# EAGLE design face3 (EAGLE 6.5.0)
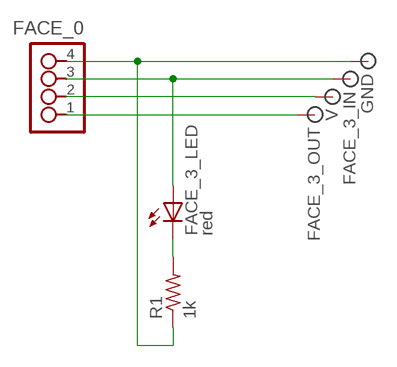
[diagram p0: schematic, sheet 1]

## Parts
FACE_0  4_PIN_HEADER  [SMT_PINS_4]
FACE_3_IN  SIGNAL  [PAD.2]
FACE_3_LED  red  LED1206  [1206]
FACE_3_OUT  SIGNAL  [PAD.2]
GND  SIGNAL  [PAD.2]
R1  1k  RESISTOR1206  [1206]
V  SIGNAL  [PAD.2]

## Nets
N$2: FACE_0.3 FACE_3_IN.P$1 FACE_3_LED.1(A)
N$3: FACE_0.2 V.P$1
N$4: FACE_0.1 FACE_3_OUT.P$1
N$5: FACE_3_LED.2(C) R1.2
N$6: FACE_0.4 GND.P$1 R1.1

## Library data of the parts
FACE_0 = ot:4_PIN_HEADER
FACE_3_IN FACE_3_OUT GND V = ot:SIGNAL: Signal
FACE_3_LED = 01_FAB_Hello:LED
R1 = 01_FAB_Hello:RESISTOR

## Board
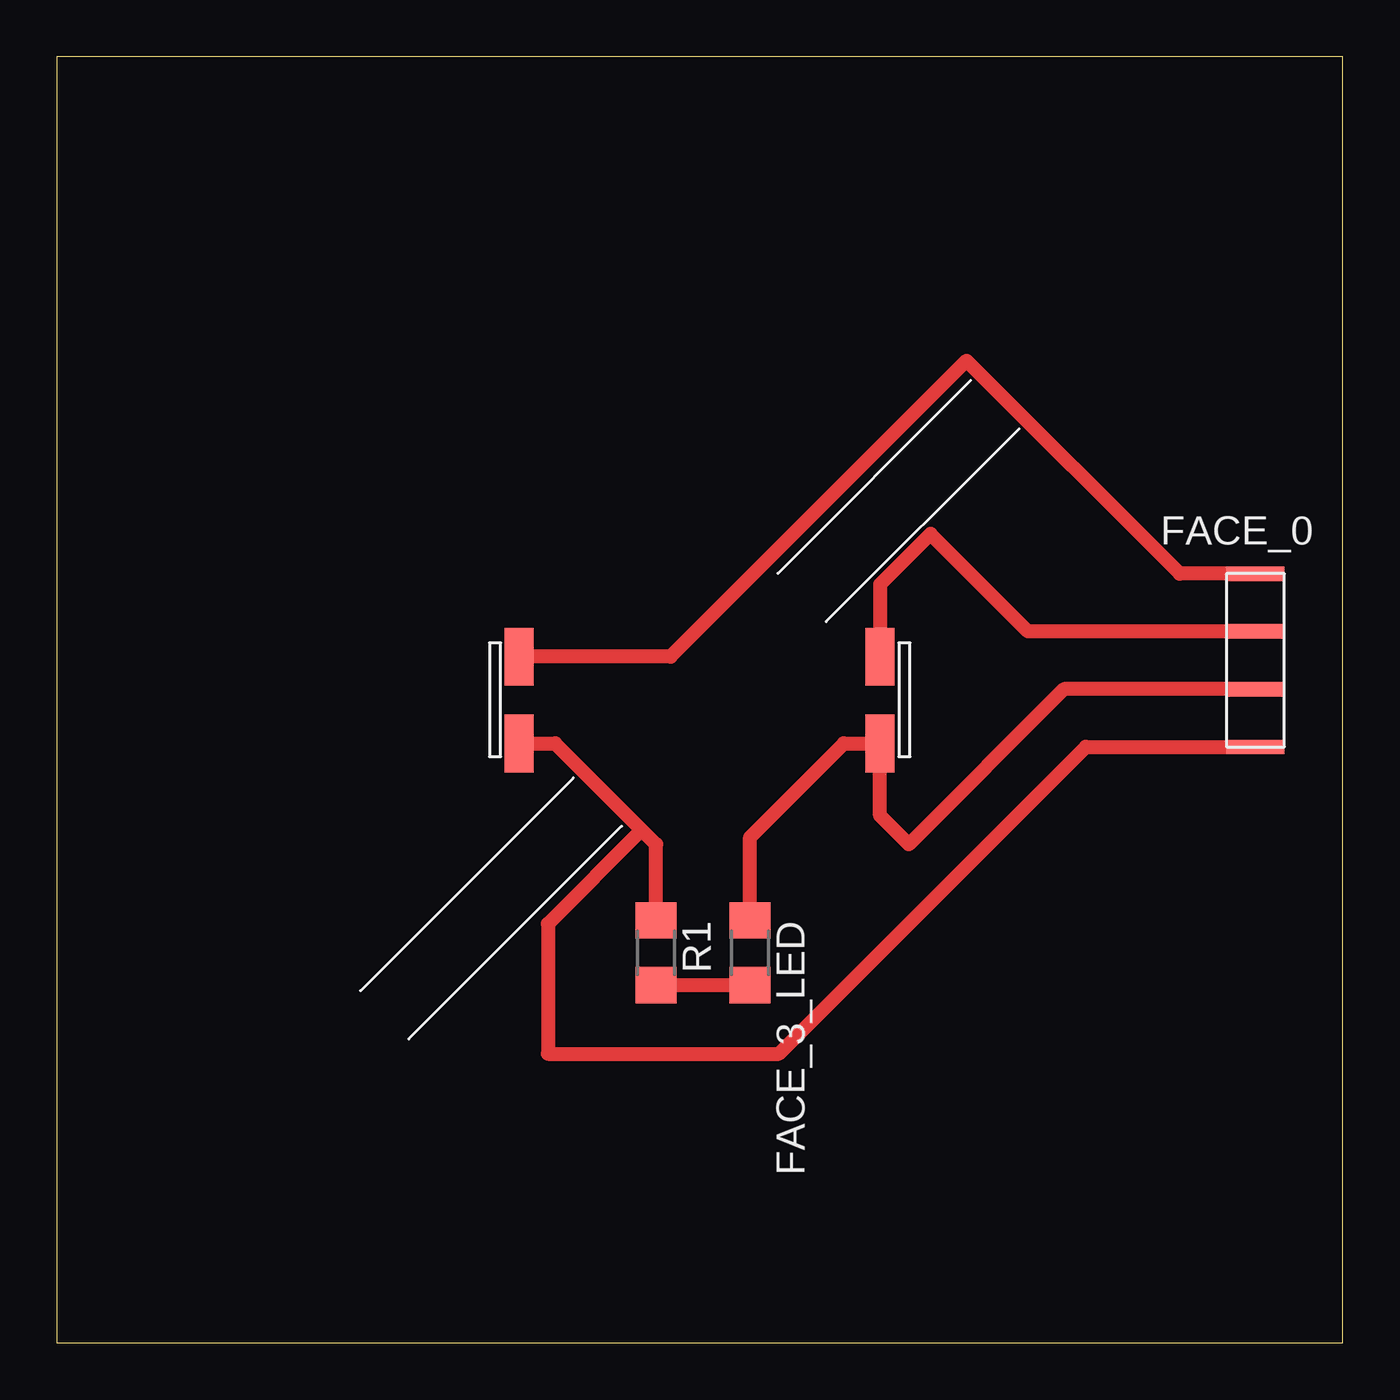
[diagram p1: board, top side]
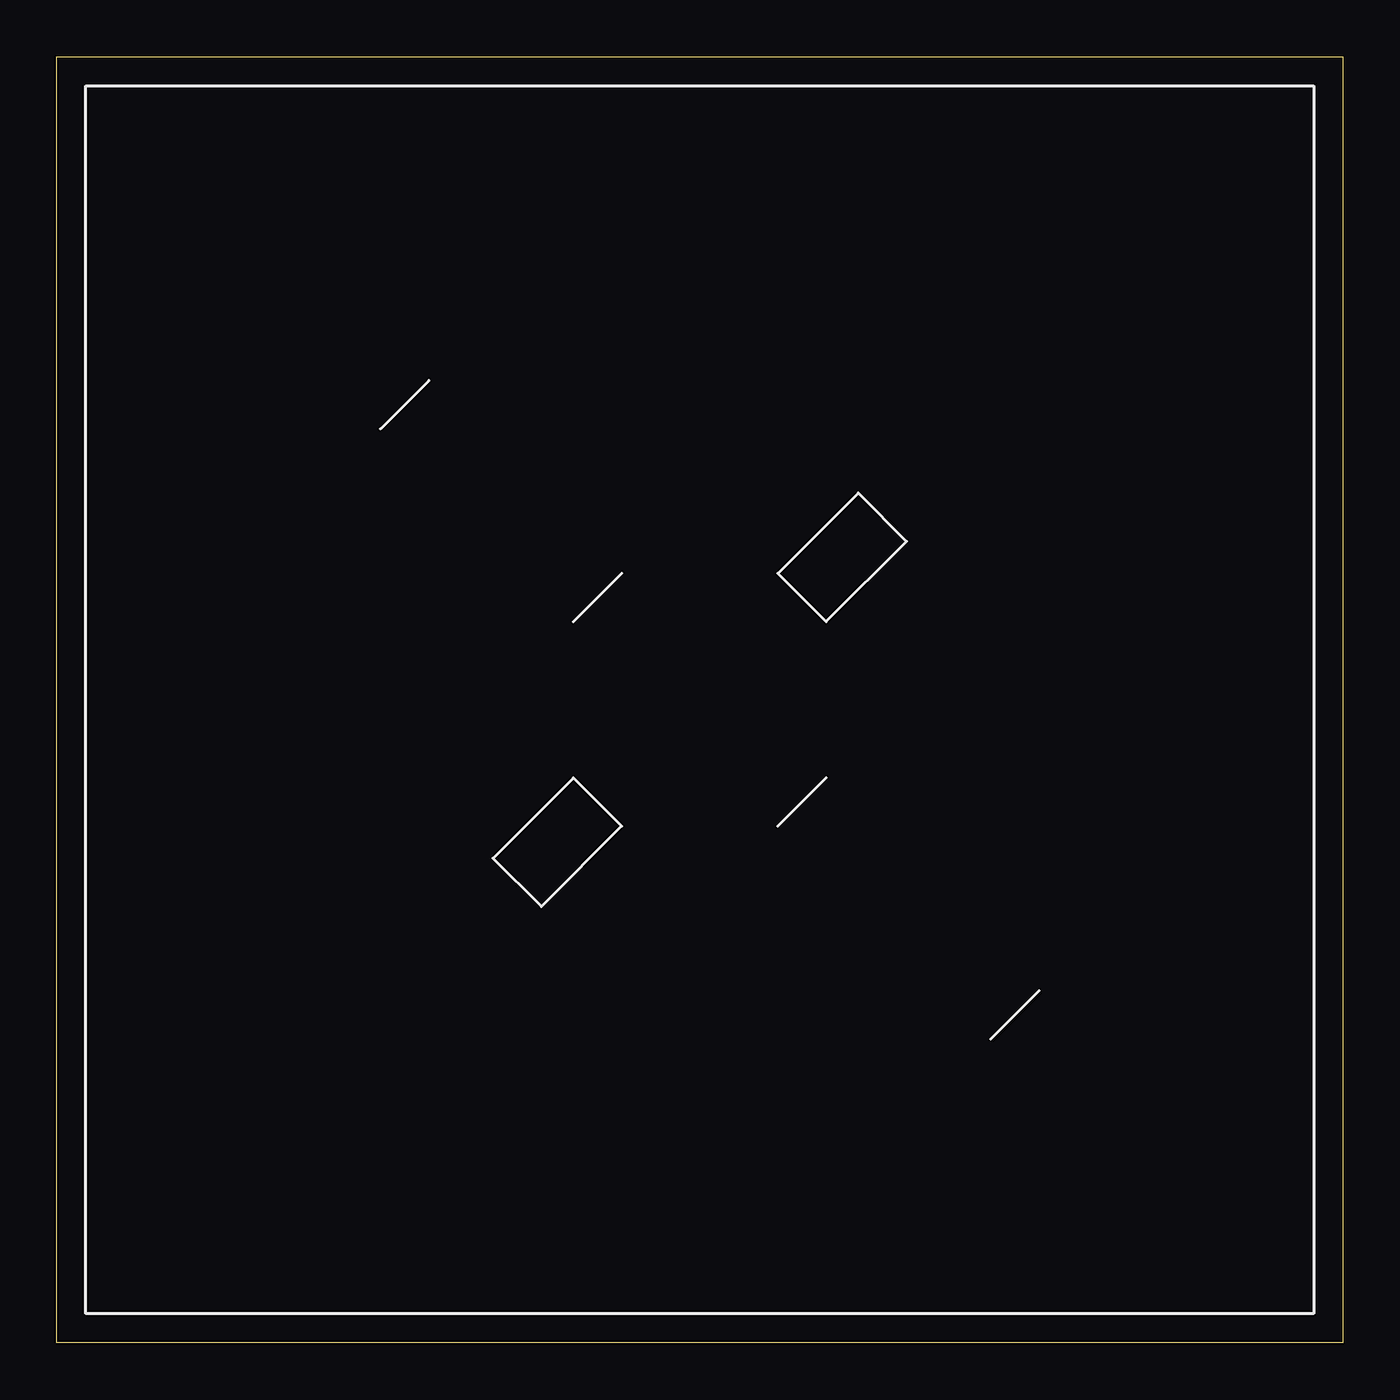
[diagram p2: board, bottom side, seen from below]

Size 56.54 x 56.54 mm. Coordinates in mm from the lower left corner, seen from the top.
Outline: 0,0 56.54,0 56.54,56.54 0,56.54 0,0
Copper layers (1*16): Top 0.035mm / dielectric 1.5mm / Bottom 0.035mm
Design rules "default": minimum track width 10mil, minimum drill 24mil, track to track 8mil, track to pad 8mil, pad to pad 8mil, via to via 8mil, smd to smd 8mil, copper to edge 40mil, drill to drill 8mil, minimum pad ring 10mil, minimum via ring 8mil, stop-mask expansion 4mil, vias tented up to drill 0mil, thermal gap 10mil

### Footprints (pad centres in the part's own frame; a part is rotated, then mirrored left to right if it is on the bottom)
SMT_PINS_4 = smd 2.54 x 0.635: 1 0,0; 2 0,2.54; 3 0,5.08; 4 0,7.62
PAD.2 = smd 2.54 x 1.27: P$1 0,0
1206 = smd 1.6 x 1.803: 1 -1.422,0; 2 1.422,0

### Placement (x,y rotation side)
FACE_0  52.7,33.81 180 top
FACE_3_IN  36.2,26.35 90 top
FACE_3_LED  30.48,17.14 270 top
FACE_3_OUT  20.32,30.16 90 top
GND  20.32,26.35 90 top
R1  26.35,17.14 270 top
U$1  [CUBE_POS]  55.27,1.27 90 top
V  36.2,30.16 90 top

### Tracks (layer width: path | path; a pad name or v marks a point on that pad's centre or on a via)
N$2
  Top 0.61: FACE_0.3 44.29,28.73 37.47,21.91 36.2,23.18 FACE_3_IN.P$1 34.61,26.35 30.48,22.23 FACE_3_LED.1
N$3
  Top 0.61: FACE_0.2 42.7,31.27 38.42,35.56 36.2,33.34 V.P$1
N$4
  Top 0.61: FACE_0.1 49.37,33.81 40.01,43.18 26.99,30.16 FACE_3_OUT.P$1
N$5
  Top 0.61: R1.2 FACE_3_LED.2
N$6
  Top 0.61: GND.P$1 21.91,26.35 25.72,22.54 | 25.72,22.54 21.59,18.41 21.59,12.7 31.75,12.7 45.24,26.19 FACE_0.4 | R1.1 26.35,21.91 25.72,22.54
